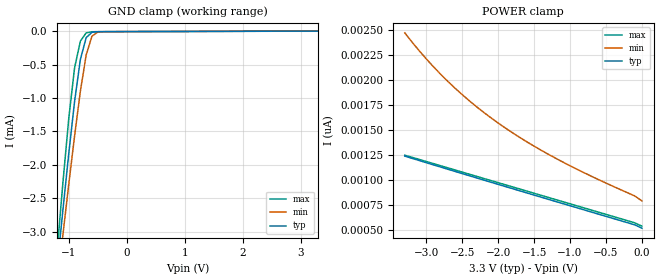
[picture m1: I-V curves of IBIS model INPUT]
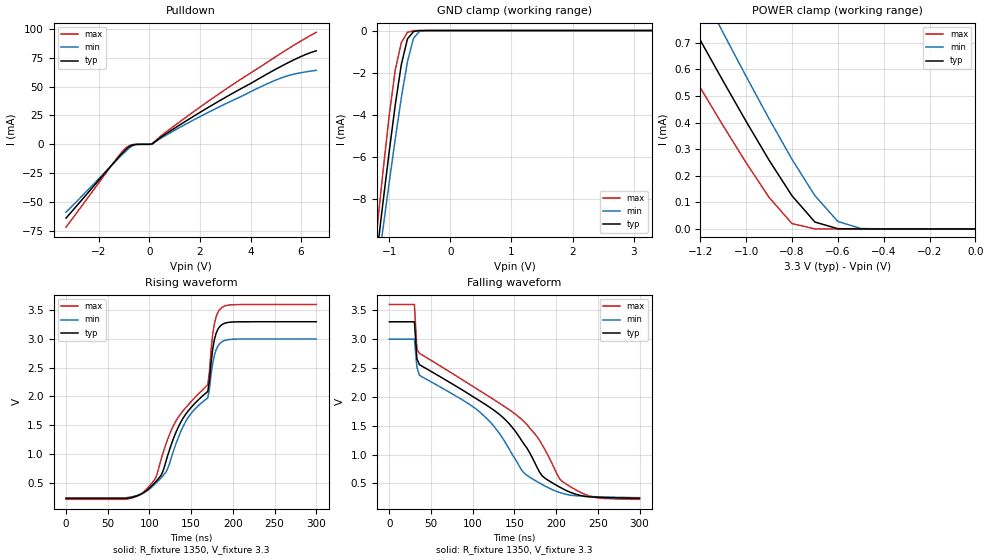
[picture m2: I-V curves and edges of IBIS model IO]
|   PERICOM SEMICONDUCTOR CORP
|   IBIS Model of PI6ULS5V9511A
|   Product Family: ULS
|   MSOP-8 (U) Package
[IBIS Ver] 3.2
[Comment char] |_char
[File Name] pi6uls5v9511a_u_33v.ibs
[File Rev] 1.0
[Source] File originated at Pericom Semiconductor Corp.
[Date] 08/30/2017
[Disclaimer] (C) Copyright PERICOM Semiconductor Corporation
   All rights reserved
  Pericom Semiconductor Corporation hereby grants the user of
  this IBIS model a non-exclusive, nontransferable license to
  use this IBIS model under the following terms.
  This IBIS model is provided on an "AS IS" basis and Pericom
  makes absolutely no warranty with respect to the information
  contained herein. PERICOM DISCLAIMS AND CUSTOMER WAIVES ALL
  WARRANTIES, EXPRESSED OR IMPLIED, INCLUDING WARRANTIES OF
  MERCHANTABILITY OR FITNESS FOR A PARTICULAR PURPOSE. The
  entire risk as to quality and performance is with the customer.
  Accordingly, in no event shall the company be liable for any
  damages, whether in contract or tort, including any lost
  profits or other incidental, consequential, exemplary, or
  punitive damages arising out of the use or application of the
  IBIS model provided in this package. Further, Pericom reserves
  the right to make changes without notice to any product herein
  to improve reliability, function, or design. Pericom does not
  convey any license under patent rights or any other intellectual
  property rights, including those of third parties.
  The user is granted this license only to use the IBIS model
  and is not granted rights to sell, load, rent, lease or license
  the IBIS model in whole or in part, or in modified form to anyone
  other than user. User may modify the IBIS model to suit its specific
  application but rights to derivative works and such modifications
  shall belong to Pericom.
  Pericom is not obligated to provide maintenance or support
  for the licensed IBIS model.
  Contact Pericom at ATTN: APPLICATION ENGINEERING / IBIS MODELS
  1545 Barber Lane Milpitas, CA 95035 USA.
[Component] PI6ULS5V9511A
[Manufacturer] Pericom Semiconductor Corp.
[Package]
| variable   typ   min   max
R_pkg   0.04200   0.03995   0.04405
L_pkg   2.30669n   2.21200n   2.40138n
C_pkg   0.21108p   0.20715p   0.21500p
[Pin] signal_name  model_name   R_pin   L_pin   C_pin
1   ENABLE   INPUT   0.04405   2.40138n   0.21500p
2   SCLOUT   IO   0.03995   2.21200n   0.20715p
3   SCLIN   IO   0.03995   2.21200n   0.20715p
4   GND   GND   0.04405   2.40138n   0.21500p
5   READY   NC   0.04405   2.40138n   0.21500p
6   SDAIN   IO   0.03995   2.21200n   0.20715p
7   SDAOUT   IO   0.03995   2.21200n   0.20715p
8   VCC   POWER   0.04405   2.40138n   0.21500p
| Models and submodels in the file (2): INPUT (Input), IO (Open_drain)
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[Model] INPUT
Model_type Input
Vinl = 990.000mV
Vinh = 2.31000V
| variable   typ   min   max
C_comp   1.640pF   1.590pF   1.690pF
[Voltage Range]   3.3000V   3.0000V   3.6000V
[POWER Clamp Reference] 3.3000V   3.0000V   3.6000V
[GND Clamp Reference]   0.0000V   0.0000V   0.0000V
[Temperature Range]   25   85   -40
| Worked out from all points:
|   GND clamp passes 1 mA (typ) near -0.89 V on its own axis
[GND Clamp]
| Voltage   I(typ)   I(min)   I(max)
-3.3V     -22.41mA   -20.33mA   -26.05mA
-1.2V     -3.522mA   -3.797mA   -3.269mA
-1.1V     -2.66mA    -3.034mA   -2.25mA
-1V       -1.827mA   -2.286mA   -1.301mA
-900mV    -1.052mA   -1.566mA   -548.2uA
-800mV    -423.5uA   -899.4uA   -150.4uA
-700mV    -98.47uA   -356.4uA   -26.64uA
-600mV    -18.3uA    -75.45uA   -9.991uA
-500mV    -9.6uA     -15.14uA   -8.807uA
3.3V      523pA      908.7pA    22.89pA
[POWER Clamp]
| Voltage   I(typ)   I(min)   I(max)
-3.3V     1.243nA    2.474nA    1.252nA
-3V       1.177nA    2.213nA    1.189nA
-2.7V     1.111nA    1.989nA    1.125nA
-2.4V     1.047nA    1.794nA    1.062nA
-2V       960.4pA    1.573nA    977.4pA
-1.7V     896.1pA    1.429nA    914.1pA
-1.3V     810.8pA    1.26nA     829.6pA
-800mV    704.7pA    1.075nA    724.1pA
-100mV    556.3pA    844.9pA    576.5pA
0V        523pA      795.8pA    542.9pA
[Model] IO
Model_type Open_drain
Vref=3.300
Rref=1.350E+03
Vmeas=1.65E+00
| variable   typ   min   max
C_comp   4.360E-12   4.350E-12   4.370E-12
[Voltage Range]   3.300E+00   3.000E+00   3.600E+00
[POWER Clamp Reference] 3.300E+00   3.000E+00   3.600E+00
[GND Clamp Reference]   0.000E+00   0.000E+00   0.000E+00
[Pullup Reference]   3.300E+00   3.000E+00   3.600E+00
[Pulldown Reference]   0.000E+00   0.000E+00   0.000E+00
[Temperature Range]   25   85   -40
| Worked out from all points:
|   slope of the pulldown table from 0 to 0.495 V, typ, clamps not added: 72.8 ohm
|   GND clamp passes 1 mA (typ) near -0.75 V on its own axis
|   POWER clamp passes 1 mA (typ) near -1.39 V on its own axis
|   rising waveform, R_fixture 1350, V_fixture 3.3: 20-80 % time 55.5ns typ, 51.6ns min, 61ns max; typ from 0.225 V to 3.3 V
|   falling waveform, R_fixture 1350, V_fixture 3.3: 20-80 % time 142ns typ, 121ns min, 161ns max; typ from 3.3 V to 0.241 V
[GND Clamp]
| Time   V(typ)   V(min)   V(max)
-3.3V     -63.95mA   -58.9mA    -71.81mA
-1.2V     -10.63mA   -11.63mA   -9.52mA
-1.1V     -8.183mA   -9.429mA   -6.716mA
-1V       -5.8mA     -7.269mA   -4.08mA
-900mV    -3.55mA    -5.173mA   -1.885mA
-800mV    -1.611mA   -3.196mA   -575.8uA
-700mV    -399.9uA   -1.479mA   -85.6uA
-600mV    -45.37uA   -362.7uA   -5.119uA
-500mV    -3.322uA   -35.76uA   -156.6nA
-300mV    -6.894nA   -162nA     -85.66pA
3.3V      83.51pA    2.672nA    81.71pA
[POWER Clamp]
| Voltage   I(typ)   I(min)   I(max)
-3.3V     4.088mA    4.535mA    3.675mA
-1.4V     1.023mA    1.241mA    822.9uA
-1.3V     865.9uA    1.071mA    676.4uA
-1.2V     709.9uA    903.6uA    531.2uA
-1.1V     555.7uA    737.5uA    388.2uA
-1V       404.6uA    574uA      249.1uA
-900mV    258.9uA    414.5uA    119uA
-800mV    124.9uA    262.2uA    20.17uA
-700mV    26.02uA    125.1uA    252.6nA
-600mV    923.4nA    28.27uA    1.759nA
-500mV    18.45nA    1.739uA    116.3pA
0V        83.51pA    116.4pA    90.66pA
[Pulldown]
| Voltage   I(typ)   I(min)   I(max)
-3.3V     -63.97mA   -58.92mA   -71.84mA
-1.3V     -13.23mA   -13.92mA   -12.54mA
-900mV    -3.852mA   -5.325mA   -2.598mA
-800mV    -2.071mA   -3.399mA   -1.273mA
-600mV    -317.6uA   -687uA     -119.3uA
100mV     180.5uA    15.15uA    426.1uA
600mV     8.28mA     7.141mA    9.7mA
2.1V      28.94mA    25.07mA    33.72mA
4.7V      61.44mA    52.8mA     71.6mA
5.6V      71.92mA    60.14mA    84.26mA
6.2V      77.95mA    62.77mA    92.11mA
6.6V      80.97mA    64.1mA     97.02mA
[Rising Waveform]
R_fixture = 1350
V_fixture = 3.3
V_fixture_min = 3.00
V_fixture_max = 3.60
| Time   V(typ)   V(min)   V(max)
0s        224.9mV    235.2mV    209.4mV
76ns      236.2mV    246mV      221.9mV
104ns     463mV      438.7mV    510mV
120ns     880.1mV    689mV      1.18V
132ns     1.382V     1.184V     1.578V
148ns     1.775V     1.666V     1.878V
170ns     2.087V     1.974V     2.205V
178ns     2.996V     2.721V     3.274V
186ns     3.24V      2.942V     3.538V
300ns     3.3V       3V         3.6V
[Falling Waveform]
R_fixture = 1350
V_fixture = 3.3
V_fixture_min = 3.00
V_fixture_max = 3.60
| Time   V(typ)   V(min)   V(max)
0s        3.3V       3.001V     3.6V
30ns      3.3V       3.001V     3.6V
33ns      2.658V     2.515V     2.823V
36ns      2.557V     2.373V     2.755V
114ns     1.878V     1.663V     2.055V
168ns     1.036V     609.1mV    1.466V
183ns     634.3mV    481.6mV    1.174V
210ns     390.7mV    316.9mV    506.3mV
246ns     261.4mV    268.9mV    259mV
300ns     240.6mV    251.6mV    222.8mV
[Ramp]
| variable   typ   min   max
dV/dt_r   1.8454E+00/5.5388E-08  1.6592E+00/5.1491E-08  2.0347E+00/6.0947E-08
dV/dt_f   1.8327E+00/1.4171E-07  1.6460E+00/1.2226E-07  2.0223E+00/1.6075E-07
R_load = 1350
